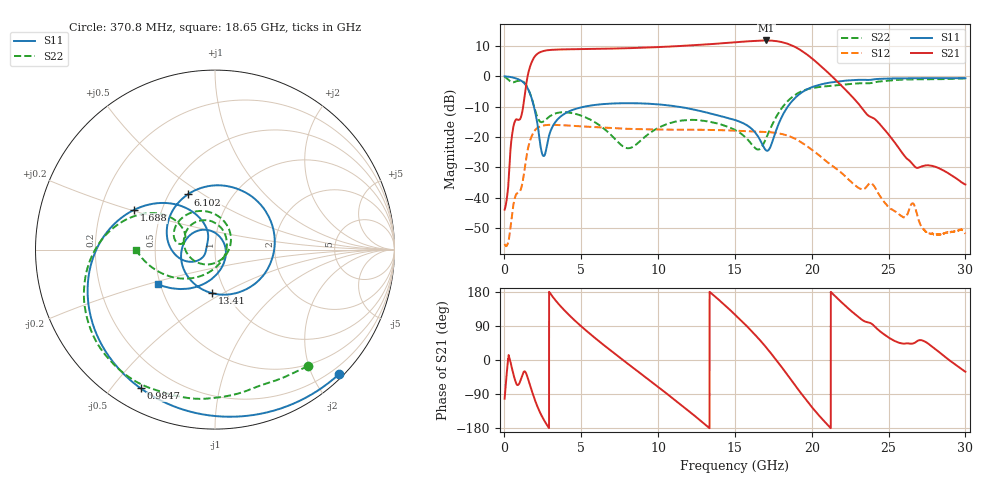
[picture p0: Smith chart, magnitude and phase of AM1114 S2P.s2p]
!Agilent Technologies,E8364B,MY43040894,A.07.50.67
!Agilent E8364B: A.07.50.67
!Date: Thursday, February 22, 2024 05:12:02
!Correction: S11(Full 2 Port(1,2))
!S21(Full 2 Port(1,2))
!S12(Full 2 Port(1,2))
!S22(Full 2 Port(1,2))
!S2P File: Measurements: S11, S21, S12, S22:
# Hz S  dB  R 50
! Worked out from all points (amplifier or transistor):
!   6401 points, 10 MHz to 30 GHz, reference 50 ohm
!   highest |S21| = 11.9 dB at 17.05 GHz (marker M1)
!   |S21| within 3 dB of that: 3.468 GHz to 19.21 GHz (15.75 GHz wide, 139 % of centre)
!   unconditionally stable (mu >= 1): 70.83 MHz to end of sweep
!   at 5.005 GHz: K = 1.26, MAG = 9.7 dB, |S12| = -16.5 dB
!   at 15.01 GHz: K = 1.27, MAG = 11.5 dB, |S12| = -17.9 dB
!   at 30 GHz: K = 212.83, MAG = -18.2 dB, |S12| = -51.9 dB
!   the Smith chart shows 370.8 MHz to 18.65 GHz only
!   S11 on the Smith chart (normalised r, x): 370.8 MHz: 0.07, -2.41; 984.7 MHz: 0.09, -0.60; 1.688 GHz: 0.35, +0.21; 6.102 GHz: 0.62, +0.43; 13.41 GHz: 0.86, -0.45; 18.65 GHz: 0.48, -0.22
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1e7  0.02 -7.8  -44.00 -102.1  -55.33 117.3  -0.16 -10.7
3.708172e8  -0.18 -45.1  -25.62 -0.7  -50.80 -133.7  -1.62 -51.4
9.84675e8  -1.14 -118.2  -14.27 -60.5  -38.05 142.0  -1.37 -117.0
1.687566e9  -5.99 153.8  3.56 -69.8  -20.88 122.3  -5.98 159.1
2.142102e9  -15.59 113.3  7.46 -122.5  -17.04 68.6  -13.41 147.1
2.924653e9  -19.20 -147.3  8.71 178.8  -16.00 9.2  -13.27 169.4
3.936816e9  -12.26 179.7  8.93 129.6  -16.16 -38.9  -11.83 140.7
5.009895e9  -10.21 146.2  9.02 88.4  -16.50 -77.5  -12.98 106.6
6.101719e9  -9.30 116.4  9.10 51.2  -16.84 -111.0  -15.84 69.8
8.008895e9  -8.85 69.8  9.32 -9.3  -17.31 -164.0  -23.71 -43.3
1.000979e10  -9.24 20.7  9.68 -71.3  -17.54 142.7  -16.98 -159.9
1.163112e10  -10.25 -25.9  10.10 -122.7  -17.61 98.9  -14.52 153.1
1.34071e10  -12.25 -93.5  10.66 177.9  -17.68 48.0  -15.05 112.4
1.5005e10  -14.40 -172.2  11.27 119.9  -17.91 -1.2  -17.68 77.5
1.608277e10  -17.28 127.6  11.67 76.4  -18.11 -35.4  -22.36 30.0
1.705275e10  -24.51 23.0  11.87 32.3  -18.33 -69.6  -20.16 -86.9
1.783062e10  -15.86 -95.2  11.55 -7.4  -18.79 -101.1  -12.14 -139.3
1.865066e10  -8.58 -148.9  10.36 -52.0  -19.96 -138.0  -7.14 -179.6
2.00049e10  -3.58 147.2  5.99 -124.1  -24.20 162.9  -3.89 127.2
2.173401e10  -1.67 90.7  -2.06 160.2  -31.03 97.6  -2.88 82.6
2.500479e10  -0.71 16.4  -19.21 59.3  -43.14 47.0  -1.37 21.6
3e10  -0.59 -74.9  -35.69 -30.7  -51.92 -96.2  -0.65 -56.7
